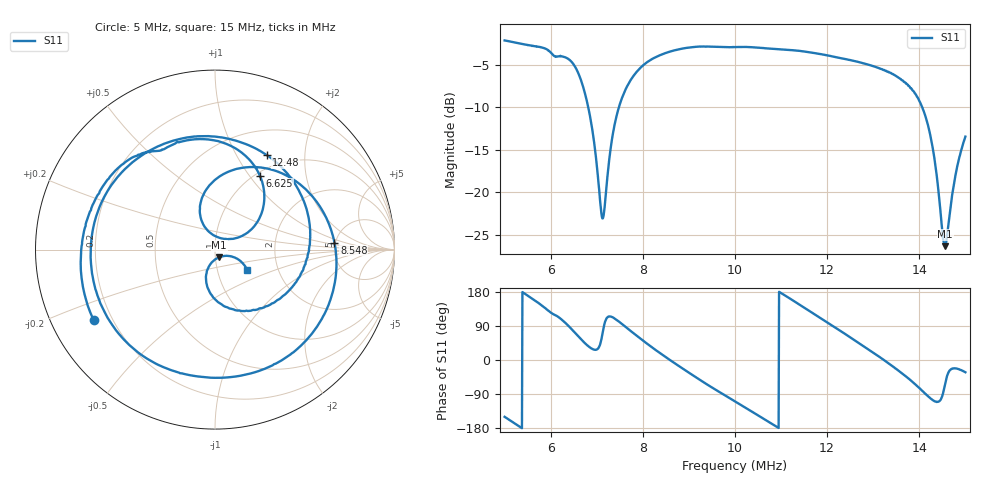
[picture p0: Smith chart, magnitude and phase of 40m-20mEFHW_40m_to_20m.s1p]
# HZ S RI R 50
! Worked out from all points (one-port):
!   1010 points, 5 MHz to 15 MHz, reference 50 ohm
!   lowest |S11| = -26.3 dB at 14.56 MHz (marker M1), VSWR 1.10, Z = 52.3 - j4.41 ohm
!   |S11| at or under -10 dB: 6.815 MHz to 7.481 MHz (666.2 kHz wide, 9.32 % of centre); 14.06 MHz to end of sweep
!   S11 on the Smith chart (normalised r, x): 5 MHz: 0.13, -0.26; 6.625 MHz: 1.05, +1.13; 8.548 MHz: 4.90, +0.68; 12.48 MHz: 0.81, +1.34; 15 MHz: 1.39, -0.33
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5000000  -0.6761 -0.3918
5307241  -0.7485 -0.0727
5614482  -0.6856 0.2399
5941545  -0.4488 0.5187
6258697  -0.1576 0.6085
6437095  0.0655 0.588
6625404  0.2496 0.4126
6883090  0.2177 0.1285
7120954  0.0276 0.0648
7338996  -0.0832 0.1958
7507483  -0.0513 0.3301
7745347  0.1139 0.4475
7983211  0.331 0.441
8548138  0.6655 0.0388
8756269  0.6707 -0.165
9390573  0.3131 -0.6482
1.000506e7  -0.2356 -0.6745
1.065918e7  -0.6519 -0.2639
1.125384e7  -0.6322 0.2631
1.188814e7  -0.2003 0.6159
1.24828e7  0.2875 0.5275
1.250263e7  0.301 0.5179
1.313693e7  0.5301 0.074
1.375141e7  0.2893 -0.3149
1.420732e7  -0.0311 -0.2342
1.456412e7  0.0239 -0.0421
1.479207e7  0.1196 -0.0488
1.50002e7  0.1797 -0.114
